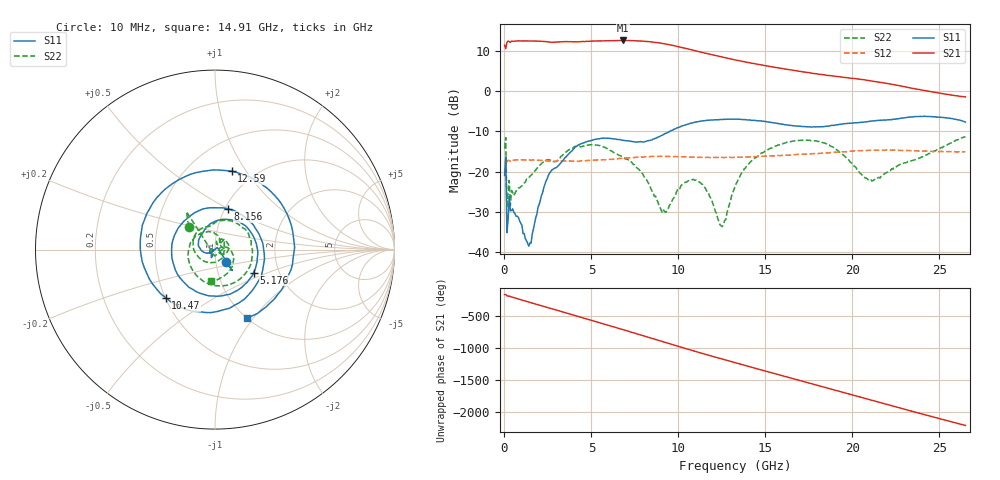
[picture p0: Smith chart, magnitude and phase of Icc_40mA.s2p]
!Keysight Technologies,N5245A,MY52451697,A.10.60.06
!Date: Thursday, May 06, 2021 15:06:22
!Correction: S11(Full 2 Port(1,4))
!S41(Full 2 Port(1,4))
!S14(Full 2 Port(1,4))
!S44(Full 2 Port(1,4))
!S2P File: Measurements: S11, S41, S14, S44:
# Hz S  dB  R 50
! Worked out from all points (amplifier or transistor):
!   401 points, 10 MHz to 26.5 GHz, reference 50 ohm
!   highest |S21| = 12.6 dB at 6.831 GHz (marker M1)
!   |S21| within 3 dB of that: start of sweep to 11.4 GHz
!   unconditionally stable (mu >= 1): start of sweep to end of sweep
!   at 4.381 GHz: K = 1.13, MAG = 12.6 dB, |S12| = -17.3 dB
!   at 13.26 GHz: K = 1.24, MAG = 9.1 dB, |S12| = -16.4 dB
!   at 26.5 GHz: K = 2.54, MAG = -0.1 dB, |S12| = -15.0 dB
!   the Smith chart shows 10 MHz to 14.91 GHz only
!   S11 on the Smith chart (normalised r, x): 10 MHz: 1.11, -0.15; 5.176 GHz: 1.48, -0.41; 8.156 GHz: 1.03, +0.50; 10.47 GHz: 0.50, -0.32; 12.59 GHz: 0.79, +0.86; 14.91 GHz: 1.00, -0.93
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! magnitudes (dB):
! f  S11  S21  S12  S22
! 10 MHz  -20.9  11.4  -19.6  -14.2
! 274.9 MHz  -26.1  12.3  -17.2  -22.2
! 407.4 MHz  -29.6  12.4  -17.1  -24.6
! 1.401 GHz  -38.5  12.4  -17.1  -21.5
! 2.593 GHz  -20.3  12.2  -17.4  -17.1
! 4.447 GHz  -13.0  12.3  -17.3  -13.8
! 5.176 GHz  -12.0  12.4  -17.1  -13.4
! 6.831 GHz  -12.2  12.6  -16.7  -16.5
! 8.156 GHz  -12.5  12.3  -16.3  -21.9
! 8.884 GHz  -11.4  12.0  -16.2  -28.4
! 9.348 GHz  -10.4  11.6  -16.2  -29.5
! 10.47 GHz  -8.3  10.5  -16.4  -22.6
! 11.4 GHz  -7.4  9.6  -16.5  -23.2
! 12.59 GHz  -7.0  8.4  -16.5  -33.1
! 13.26 GHz  -6.9  7.7  -16.4  -23.7
! 13.92 GHz  -7.1  7.2  -16.4  -18.7
! 14.91 GHz  -7.5  6.4  -16.2  -15.2
! 17.69 GHz  -8.9  4.4  -15.5  -12.3
! 18.95 GHz  -8.5  3.7  -15.2  -14.1
! 21 GHz  -7.5  2.6  -14.7  -22.2
! 22.13 GHz  -7.1  1.8  -14.6  -19.7
! 26.5 GHz  -7.7  -1.4  -15.0  -11.3
